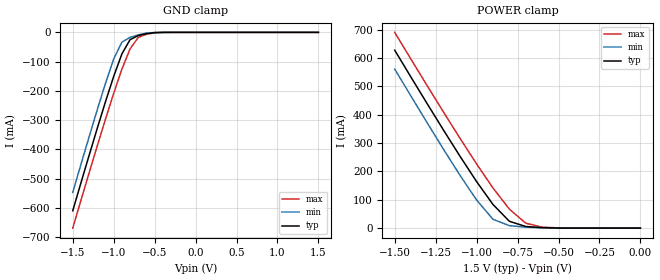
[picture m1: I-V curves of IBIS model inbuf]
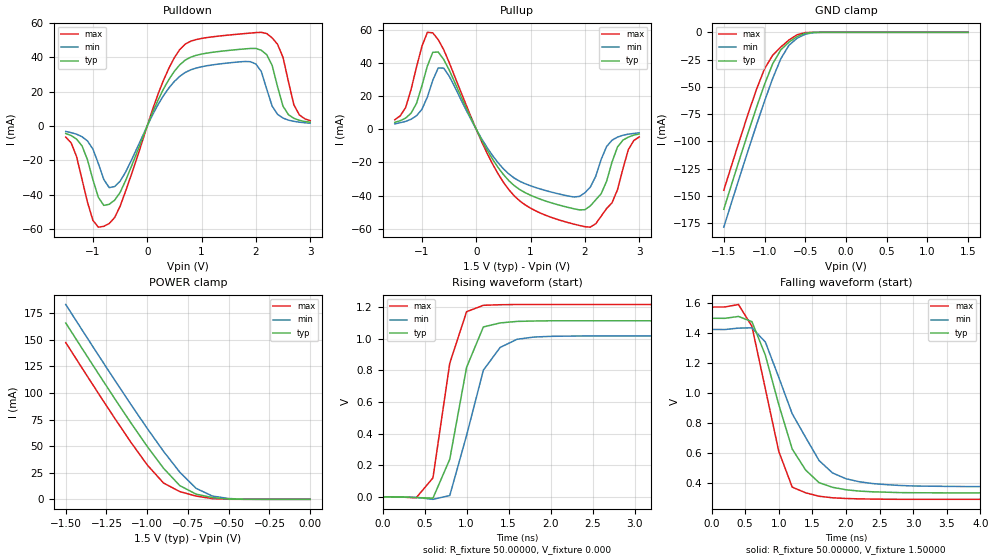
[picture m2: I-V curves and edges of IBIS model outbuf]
| IBIS file ics651_1p5.ibs created by s2ibis2 version 1.2
| North Carolina State University Electronics Research Laboratory  1995
[IBIS ver]   2.1
[File name]   ics651_1p5.ibs
[File Rev]   1.0
[Date]   May 12, 2006
[Source]   IDT
[Notes]   1. Temp typ=25C, min=+85C, max=-40C 2. Ramp rates based on 50
   ohm load
[Disclaimer] READ THESE TERMS AND CONDITIONS CAREFULLY BEFORE USING THIS
   IBIS MODEL. BY USING THIS IBIS MODEL, YOU ARE ACCEPTING AND
   AGREEING TO THESE TERMS AND CONDITIONS OF USE. Integrated
   Device Technology, Inc. ("IDT") hereby grants the user of this
   IBIS model ("User") a non-exclusive, nontransferable license
   to use this IBIS model under the following terms: The User is
   granted this license only to use the IBIS model for
   demonstration purposes only and is not granted rights to sell,
   copy (except as needed to run the IBIS model), rent, lease or
   sub-license (except for demonstration) the IBIS model in whole
   or in part, or in modified form to anyone. The User may modify
   the IBIS model to suit its specific applications, but rights
   to derivative works and such modifications shall belong to
   IDT. THIS IBIS MODEL IS PROVIDED ON AN AS IS" BASIS AND IDT
   MAKES ABSOLUTELY NO WARRANTY WITH RESPECT TO THE INFORMATION
   CONTAINED HEREIN. IDT DISCLAIMS AND USER WAIVES ALL
   WARRANTIES, EXPRESS AND IMPLIED, INCLUDING WARRANTIES OF
   MERCHANTABILITY AND FITNESS FOR A PARTICULAR PURPOSE. THE
   ENTIRE RISK AS TO QUALITY AND PERFORMANCE IS WITH THE USER
   ACCORDINGLY, IN NO EVENT SHALL IDT BE LIABLE FOR ANY DIRECT OR
   INDIRECT DAMAGES, WHETHER IN CONTRACT OR TORT, INCLUDING ANY
   LOST PROFITS OR OTHER INCIDENTAL, CONSEQUENTIAL, EXEMPLARY, OR
   PUNITIVE DAMAGES ARISING OUT OF THE USE OR APPLICATION OF THE
   IBIS MODEL, WHETHER OR NOT IDT HAD NOTICE OF SUCH DAMAGES. IDT
   reserves the right to make changes without notice to any
   product herein to improve reliability, function, or design.
   IDT does not convey any license under patent rights or any
   other intellectual property rights, including those of third
   parties. IDT is not obligated to provide maintenance or
   support for the licensed IBIS model.
   **************************************** This model is for
   ICS651 IDT Clock ****************************************
[Copyright]   Copyright 2006, Integrated Device Technology, Inc. All rights
   reserved.
|   Component ICS651
[Component]   ICS651
[Manufacturer]   Integrated Device Technology Inc.
[Package]
| variable   typ   min   max
R_pkg   40.00000m   35.00000m   45.00000m
L_pkg   1.65000nH   1.35000nH   1.95000nH
C_pkg   0.24000pF   0.14000pF   0.34000pF
[Pin]  signal_name   model_name   R_pin   L_pin   C_pin
1   ICLK   inbuf
2   Q1   outbuf
3   Q2   outbuf
4   Q3   outbuf
5   Q4   outbuf
6   GND   GND
7   VDD   POWER
8   OE   inbuf
| Models and submodels in the file (2): inbuf (Input), outbuf (3-state)
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|   Model inbuf
[Model]   inbuf
Model_type   Input
Vinl =  0.63000V
Vinh =  1.17000V
C_comp   5.50000pF   5.00000pF   6.00000pF
[Temperature Range]   25.00000   85.00000   -40.00000
[Voltage Range]   1.50000V   1.42500V   1.57500V
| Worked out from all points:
|   GND clamp passes 1 mA (typ) near -0.50 V on its own axis
|   POWER clamp passes 1 mA (typ) near -0.55 V on its own axis
[GND_clamp]
| voltage   I(typ)   I(min)   I(max)
-1.5V     -610mA     -547.2mA   -669.3mA
-1.2V     -327.6mA   -264mA     -387.6mA
-1.1V     -237mA     -174mA     -296.6mA
-1V       -150.5mA   -91.29mA   -208.5mA
-900mV    -73.81mA   -33.43mA   -126.1mA
-800mV    -24.96mA   -17.14mA   -56.58mA
-700mV    -10.95mA   -8.596mA   -17.39mA
-600mV    -4.469mA   -2.509mA   -6.337mA
-400mV    -79.64uA   -11.48uA   -290uA
1.5V      766pA      -656.7nA   507.7nA
[POWER_clamp]
| voltage   I(typ)   I(min)   I(max)
-1.5V     627.6mA    561mA      690.5mA
-1.2V     343.8mA    276.2mA    407.4mA
-1.1V     252.3mA    185mA      315.6mA
-1V       164.1mA    99.28mA    226.4mA
-900mV    83.43mA    31.03mA    141.7mA
-800mV    24.16mA    8.748mA    66.96mA
-700mV    5.75mA     3.409mA    17.53mA
-600mV    1.75mA     719.6uA    3.531mA
-400mV    29.79uA    6.711uA    115.3uA
0V        766pA      84.23pA    22.02nA
|   Model outbuf
[Model]   outbuf
Model_type   3-state
Polarity   Non-Inverting
Enable   Active-Low
Vmeas =  0.75000V
Rref = 50.00000
Vref =  0.000V
C_comp   5.50000pF   5.00000pF   6.00000pF
[Temperature Range]   25.00000   85.00000   -40.00000
[Voltage Range]   1.50000V   1.42500V   1.57500V
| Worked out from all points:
|   slope of the pulldown table from 0 to 0.225 V, typ, clamps not added: 13.4 ohm
|   slope of the pullup table from 0 to 0.225 V, typ, clamps not added: 16.2 ohm
|   GND clamp passes 1 mA (typ) near -0.50 V on its own axis
|   POWER clamp passes 1 mA (typ) near -0.55 V on its own axis
|   rising waveform, R_fixture 50.00000, V_fixture 0.000: 20-80 % time 269ps typ, 315ps min, 245ps max; typ from 0 V to 1.11 V
|   falling waveform, R_fixture 50.00000, V_fixture 1.50000: 20-80 % time 496ps typ, 647ps min, 392ps max; typ from 1.5 V to 0.331 V
[Pulldown]
| voltage   I(typ)   I(min)   I(max)
-1.5V     -4.4mA     -3.2mA     -6.5mA
-1.2V     -11.61mA   -6.3mA     -31.21mA
-900mV    -41.61mA   -21.87mA   -59.01mA
-700mV    -45.68mA   -35.95mA   -56.9mA
-500mV    -38.82mA   -32.24mA   -46.85mA
300mV     21.56mA    17.71mA    26.67mA
800mV     40.1mA     32.72mA    49.42mA
1.9V      45.19mA    37.47mA    54.17mA
2.2V      41.53mA    21.5mA     53.91mA
2.6V      6.58mA     3.4mA      25.84mA
2.8V      3.3mA      2.2mA      6.47mA
3V        2.2mA      1.6mA      3.1mA
[Pullup]
| voltage   I(typ)   I(min)   I(max)
-1.5V     4.2mA      3.3mA      5.8mA
-1.3V     6.8mA      4.8mA      13.15mA
-1.1V     15.66mA    8.19mA     37.62mA
-900mV    38.26mA    19.5mA     58.62mA
-800mV    46.54mA    29.65mA    58.3mA
-600mV    42.27mA    37.02mA    48.21mA
600mV     -31.02mA   -26.97mA   -36.47mA
1.8V      -48.02mA   -40.89mA   -57.3mA
2.1V      -46.28mA   -34.91mA   -59.12mA
2.5V      -19.75mA   -6.58mA    -44.38mA
2.8V      -4.7mA     -2.9mA     -12.28mA
3V        -2.8mA     -2.1mA     -4.6mA
[GND_clamp]
| voltage   I(typ)   I(min)   I(max)
-1.5V     -162.1mA   -178.5mA   -144.7mA
-1.2V     -91.59mA   -107.9mA   -74.39mA
-1.1V     -69.05mA   -85.13mA   -52.51mA
-1V       -47.67mA   -63.05mA   -33.38mA
-900mV    -28.89mA   -42.27mA   -21.03mA
-800mV    -16.04mA   -24.21mA   -13.46mA
-700mV    -8.94mA    -11.82mA   -7.05mA
-600mV    -3.886mA   -5.387mA   -2.229mA
-500mV    -872.3uA   -1.753mA   -231uA
-400mV    -76.24uA   -282.3uA   -7.635uA
-300mV    -3.678uA   -25.68uA   -126.1nA
1.5V      766pA      52.8nA     72.12pA
[POWER_clamp]
| voltage   I(typ)   I(min)   I(max)
-1.5V     165.9mA    183.3mA    147.5mA
-1.2V     94.87mA    112.3mA    76.35mA
-1.1V     71.9mA     89.23mA    53.65mA
-1V       49.75mA    66.73mA    32.37mA
-900mV    29.23mA    45.17mA    15.35mA
-800mV    12.89mA    25.51mA    7.266mA
-700mV    4.877mA    10.33mA    3.05mA
-600mV    1.627mA    3.084mA    683.2uA
-500mV    287.7uA    748.1uA    58.05uA
-400mV    26.3uA     111.6uA    2.376uA
0V        766pA      22.02nA    84.4pA
[Ramp]
| variable   typ   min   max
dV/dt_r   0.66840/0.22536n   0.61080/0.29010n   0.73020/0.18275n
dV/dt_f   0.70140/0.46379n   0.63150/0.58217n   0.77226/0.35502n
R_load = 50.00000
[Rising Waveform]
R_fixture = 50.00000
V_fixture = 0.000
V_fixture_min = 0.000
V_fixture_max = 0.000
| time   V(typ)   V(min)   V(max)
0s        0V         0V         0V
400ps     -4.404mV   -3.343mV   -6.376mV
600ps     -8.243mV   -15.61mV   120.2mV
800ps     238.2mV    8.28mV     845.2mV
1ns       819.3mV    388.8mV    1.171V
1.2ns     1.075V     801.6mV    1.212V
1.4ns     1.101V     945.4mV    1.216V
1.6ns     1.11V      996.9mV    1.217V
1.8ns     1.113V     1.011V     1.217V
10ns      1.114V     1.018V     1.217V
[Falling Waveform]
R_fixture = 50.00000
V_fixture = 1.50000
V_fixture_min = 1.42500
V_fixture_max = 1.57500
| time   V(typ)   V(min)   V(max)
0s        1.5V       1.425V     1.575V
400ps     1.512V     1.434V     1.592V
600ps     1.477V     1.436V     1.446V
800ps     1.253V     1.341V     1.028V
1ns       921.5mV    1.104V     608.8mV
1.2ns     624.1mV    860.4mV    369.6mV
1.4ns     483.7mV    702.1mV    331.6mV
1.8ns     368.4mV    464.2mV    298.2mV
2.4ns     338.1mV    393.2mV    289.6mV
10ns      331mV      372.5mV    287.9mV
